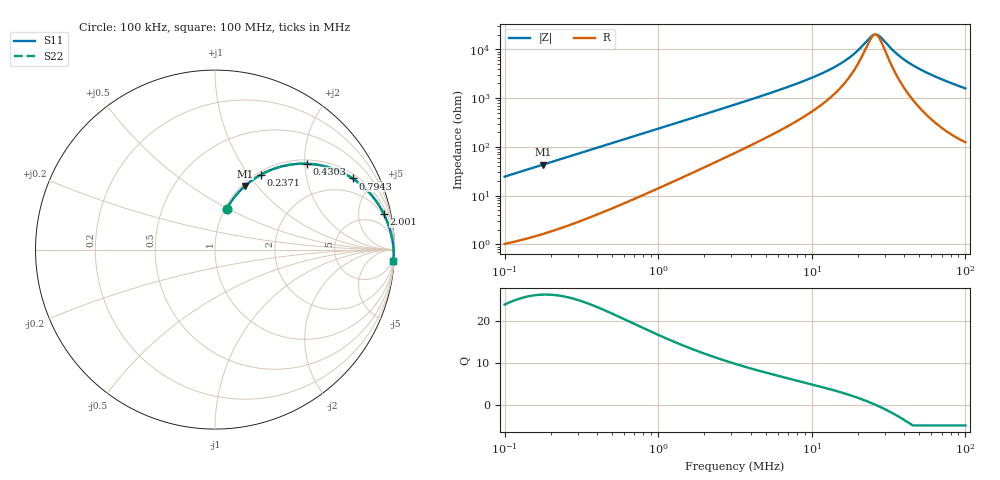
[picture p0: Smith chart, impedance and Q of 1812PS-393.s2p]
# MHz S MA R 50
!Freq  MagS11  AngS11  MagS21  AngS21  MagS12  AngS12  MagS22  AngS22
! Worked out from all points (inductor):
!   801 points, 100 kHz to 100 MHz, reference 50 ohm
!   read as one part in series: L = 38.9 uH near 103.5 kHz
!   highest Q = 26.3 at 178.3 kHz (marker M1), where L = 38.7 uH
!   self-resonance near 25.78 MHz
!   S11 on the Smith chart (normalised r, x): 100 kHz: 1.02, +0.49; 237.1 kHz: 1.04, +1.15; 430.3 kHz: 1.09, +2.06; 794.3 kHz: 1.20, +3.75; 2.001 MHz: 1.76, +9.31; 100 MHz: 3, -31
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0.1  0.2363 74.0  0.9619 -13.7  0.9619 -13.7  0.2363 74.0
0.1783405  0.3923 64.7  0.9051 -23.1  0.9051 -23.1  0.3923 64.7
0.2371374  0.4894 58.5  0.8535 -29.3  0.8535 -29.3  0.4894 58.5
0.3180534  0.5961 51.1  0.7792 -36.6  0.7792 -36.6  0.5961 51.1
0.4302789  0.702 43.0  0.6821 -44.5  0.6821 -44.5  0.702 43.0
0.7943282  0.8635 27.3  0.4595 -59.6  0.4595 -59.6  0.8635 27.3
1.002882  0.9017 22.4  0.3816 -64.2  0.3816 -64.2  0.9017 22.4
2.001013  0.9619 11.8  0.206 -73.5  0.206 -73.5  0.9619 11.8
3.162278  0.9777 7.6  0.1326 -76.6  0.1326 -76.6  0.9777 7.6
6.255327  0.9882 3.7  0.06588 -77.8  0.06588 -77.8  0.9882 3.7
10.05773  0.9917 2.1  0.0377 -76.2  0.0377 -76.2  0.9917 2.1
13.37365  0.993 1.4  0.02497 -73.1  0.02497 -73.1  0.993 1.4
16.73979  0.9939 0.9  0.01641 -67.7  0.01641 -67.7  0.9939 0.9
19.38653  0.9943 0.6  0.0114 -60.0  0.0114 -60.0  0.9943 0.6
23.85064  0.9949 0.2  0.005776 -27.6  0.005776 -27.6  0.9949 0.2
25.3367  0.995 0.0  0.00502 -6.9  0.00502 -6.9  0.995 0.0
27.62167  0.9952 -0.1  0.005365 26.1  0.005365 26.1  0.9952 -0.1
31.71393  0.9954 -0.4  0.008527 57.2  0.008527 57.2  0.9954 -0.4
38.34864  0.9956 -0.8  0.01474 72.3  0.01474 72.3  0.9956 -0.8
48.83711  0.9956 -1.4  0.02402 78.9  0.02402 78.9  0.9956 -1.4
67.80317  0.9951 -2.2  0.03922 81.7  0.03922 81.7  0.9951 -2.2
100  0.9931 -3.6  0.06289 81.9  0.06289 81.9  0.9931 -3.6
